TYPE E_AnalysisIDs :
(
	(* analysis chain *)
	eID_Source_DFT := 1,
	eID_Source_Spectrum,
	(* sparse algorithms *)
	eID_SparseSpectrum_DFT,
	eID_SparseSpectrum_Magnitude,
	eID_SparseSpectrum_Power,
	(* reference algorithms *)
	eID_RealFFT,
	eID_MagnitudeSpectrum,
	eID_PowerSpectrum,
	(* sinks *)
	eID_Sink_DFT,
	eID_Sink_Magnitude,
	eID_Sink_Power,
	eID_Sink_RealFFT,
	eID_Sink_MagnitudeSpectrum,
	eID_Sink_PowerSpectrum
) UDINT;
END_TYPE
